FUNCTION_BLOCK AssignableDigitalInputChannel implements I_DigitalInput
VAR
	digitalInput : I_DigitalInput;
END_VAR

METHOD PUBLIC ChangeDigitalInput
VAR_INPUT
	DigitalInput : I_DigitalInput;
END_VAR
IF DigitalInput <> 0 THEN
	THIS^.digitalInput := DigitalInput;
END_IF
END_METHOD

METHOD FB_init : BOOL
VAR_INPUT
	bInitRetains : BOOL; // if TRUE, the retain variables are initialized (warm start / cold start)
	bInCopyCode : BOOL;  // if TRUE, the instance afterwards gets moved into the copy code (online change)
	DigitalInput : I_DigitalInput;
END_VAR
this^.digitalInput := DigitalInput;
END_METHOD

PROPERTY PUBLIC State : BOOL
GET
State := digitalInput.State;
END_GET
END_PROPERTY

END_FUNCTION_BLOCK
